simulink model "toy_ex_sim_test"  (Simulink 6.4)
settings: Solver=ode4  StartTime=0.0  StopTime=simtid  RelTol=1e-5
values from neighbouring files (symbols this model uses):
  den_G1 = [-1 1]    [bounds.m]    (also in toy_ex_nytt_system.m; toy_ex_nytt_system_without_noise.m; toy_ex_nytt_system_with_disturbance.m; toy_ex_nytt_system_with_measure_noise.m)
  den_G2 = [-1 1]    [bounds.m]    (also in toy_ex_nytt_system.m; toy_ex_nytt_system_without_noise.m; toy_ex_nytt_system_with_disturbance.m; toy_ex_nytt_system_with_measure_noise.m)
  K_indre = 10    [real_ex_linkomb_W_and_DP.m]    (also in real_ex_linkomb_W_and_RHOT.m = 5; toy_ex_nytt_system.m = 50; toy_ex_nytt_system_without_noise.m = 20; toy_ex_nytt_system_with_disturbance.m = 50)
  K_ytre = 0.01    [real_ex_linkomb_W_and_DP.m]    (also in real_ex_linkomb_W_and_RHOT.m; toy_ex_nytt_system.m = 0.1; toy_ex_nytt_system_without_noise.m = 0.1; toy_ex_nytt_system_with_disturbance.m = 0.1)
  num_G1 = 5*[-1.5 1]    [bounds.m]    (also in toy_ex_nytt_system.m; toy_ex_nytt_system_without_noise.m; toy_ex_nytt_system_with_disturbance.m; toy_ex_nytt_system_with_measure_noise.m)
  num_G2 = 5*[-0.5 1]    [bounds.m]    (also in toy_ex_nytt_system.m; toy_ex_nytt_system_without_noise.m; toy_ex_nytt_system_with_disturbance.m; toy_ex_nytt_system_with_measure_noise.m)

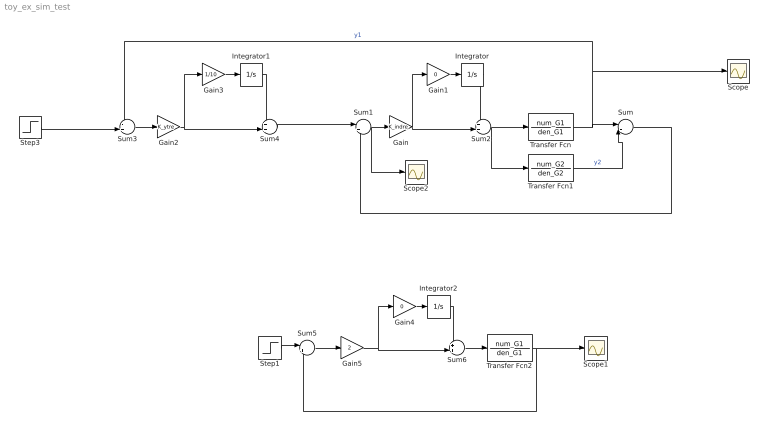
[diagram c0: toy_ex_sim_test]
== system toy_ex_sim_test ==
  Gain : Gain  Gain=K_indre
  Gain1 : Gain  Gain=0
  Gain2 : Gain  Gain=K_ytre
  Gain3 : Gain  Gain=1/10
  Gain4 : Gain  Gain=0
  Gain5 : Gain  Gain=2
  Integrator : Integrator
  Integrator1 : Integrator
  Integrator2 : Integrator
  Scope : Scope
  Scope1 : Scope
  Scope2 : Scope
  Step1 : Step  SampleTime=0
  Step3 : Step  SampleTime=0
  Sum : Sum  Inputs=|+-
  Sum1 : Sum  Inputs=|+-
  Sum2 : Sum  Inputs=++|
  Sum3 : Sum  Inputs=-+|
  Sum4 : Sum  Inputs=++|
  Sum5 : Sum  Inputs=|+-
  Sum6 : Sum  Inputs=++|
  Transfer Fcn : TransferFcn  Numerator=num_G1  Denominator=den_G1
  Transfer Fcn1 : TransferFcn  Numerator=num_G2  Denominator=den_G2
  Transfer Fcn2 : TransferFcn  Numerator=num_G1  Denominator=den_G1
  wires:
  Sum1/1 -> Gain/1, Scope2/1
  Sum/1 -> Sum1/2
  Gain1/1 -> Integrator/1
  Gain/1 -> Gain1/1, Sum2/2
  Transfer Fcn1/1 -> Sum/2  "y2"
  Transfer Fcn/1 -> Sum/1, Scope/1, Sum3/1  "y1"
  Integrator/1 -> Sum2/1
  Sum2/1 -> Transfer Fcn/1, Transfer Fcn1/1
  Sum3/1 -> Gain2/1
  Gain3/1 -> Integrator1/1
  Integrator1/1 -> Sum4/1
  Gain2/1 -> Sum4/2, Gain3/1
  Sum4/1 -> Sum1/1
  Gain4/1 -> Integrator2/1
  Integrator2/1 -> Sum6/1
  Sum5/1 -> Gain5/1
  Gain5/1 -> Sum6/2, Gain4/1
  Sum6/1 -> Transfer Fcn2/1
  Transfer Fcn2/1 -> Sum5/2, Scope1/1
  Step1/1 -> Sum5/1
  Step3/1 -> Sum3/2
